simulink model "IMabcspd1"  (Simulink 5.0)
settings: Solver=ode45  StartTime=0.0  StopTime=4.0  RelTol=1e-3
InitFcn:
  | imparamspd1
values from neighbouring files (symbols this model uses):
  Bm = 0.10    (= 0.1)    [IMabc2.m]    (also in imabcparam.m = 0.01; IMabcrun0.m = 0.01; IMabcrun1.m = 0.001; IMcur0.m = 1e-06)
  gam = 2*pi/3    (= 2.09439510239)    [IMabc2.m]    (also in IMabcf0.m; IMabcf1.m; imabcparam.m; IMabcrun0.m)
  J = 0.02    [imabcparam.m]    (also in IMabcrun0.m; IMabcrun1.m; imdefSIvec1.m = 0.03)
  Lm1 = 2/3*Lm    [IMabcf0.m]    (also in IMabcf1.m; imabcparam.m = 0.0564666666667; IMabcrun0.m = 0.0564666666667; IMabcrun1.m = 0.0564666666667)
  Lrr = [Lr   -Lm/2 -Lm/2    [IMabc2.m]    (also in IMabcf0.m = [Lr   -Lm1/2 -Lm1/2; IMabcf1.m = [Lr   -Lm1/2 -Lm1/2)
  Lss = [Ls   -Lm/2 -Lm/2    [IMabc2.m]    (also in IMabcf0.m = [Ls   -Lm1/2 -Lm1/2; IMabcf1.m = [Ls   -Lm1/2 -Lm1/2)
  nsync = 120*freq0/p    (= 1800)    [imabcparam.m]
  p = cos(beta-alpha)    [abcRwdg.m]    (also in alternator.m = 0:pi/20:2*pi; altwdgs.m = 0:pi/20:2*pi; brushlessdcB.m = 0:pi/100:2*pi; brushlessdcnew.m = 0:pi/100:2*pi)
  R = str2num(get(h,'string'))    [acttrcalc1.m]    (also in IMabc2.m = diag([Rs Rs Rs Rr Rr Rr]); IMabcf0.m = diag([Rs Rs Rs Rr Rr Rr]); IMabcf1.m = diag([Rs Rs Rs Rr Rr Rr]); IMcurf0.m = diag([Rs Rs Rr Rr]))
  Vm = Vll*sqrt(2/3)    [imabcparam.m]
  wo = 2*pi*freq0    [calc0.m]    (also in IMabc2.m = 376.991118431; imabcparam.m = 376.991118431; IMabcrun0.m = 376.991118431; IMabcrun1.m = 376.991118431)
undefined symbols (not defined in the file or in its folder): TL1
libraries: simulink x9

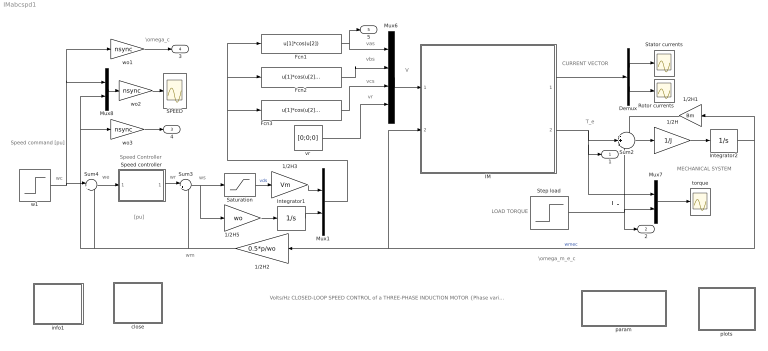
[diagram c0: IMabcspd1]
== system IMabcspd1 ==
  note: LOAD TORQUE
  note: T_L
  note: Volts/Hz CLOSED-LOOP SPEED CONTROL of a THREE-PHASE INDUCTION MOTOR {Phase variable model}
  note: T_e
  note: I
  note: MECHANICAL SYSTEM
  note: \omega_m_e_c
  note: CURRENT VECTOR
  note: V
  note: wr
  note: we
  note: wm
  note: vas
  note: vbs
  note: vcs
  note: vr
  note: Speed command [pu]
  note: \omega_c
  note: [pu]
  note: ws
  note: Speed Controller
  note: wc
  1/2H : Gain  Gain=1/J
  1/2H1 : Gain  Orientation=left  Gain=Bm
  1/2H2 : Gain  Orientation=left  Gain=0.5*p/wo
  1/2H3 : Gain  Gain=Vm
  1/2H5 : Gain  Gain=wo
  Demux : Demux  Outputs=2
  Fcn1 : Fcn  Expr=u[1]*cos(u[2])
  Fcn2 : Fcn  Expr=u[1]*cos(u[2]-gam)
  Fcn3 : Fcn  Expr=u[1]*cos(u[2]+gam)
  IM : Subsystem
  Integrator1 : Integrator
  Integrator2 : Integrator
  Mux1 : Mux  Inputs=2
  Mux6 : Mux
  Mux7 : Mux  Inputs=2
  Mux8 : Mux  Inputs=2
  Rotor currents : Scope
  SPEED : Scope
  Saturation : Saturate  UpperLimit=1  LowerLimit=-1
  Speed controller : Subsystem  mask{Kp=0.6, Ki=5.6, sat=0.03}
      mask prompts: Kp "Proportional gain (Kp)"; Ki "Integral gain (Ki)"; sat "Saturation limit [pu]"
      mask help: Proportional-Integral Speed Controller
  Stator currents : Scope
  Step load : Step  Time=2  Before=0.0  After=TL1  SampleTime=0
  Sum2 : Sum  Inputs=-+-
  Sum3 : Sum  Inputs=|++
  Sum4 : Sum  Inputs=|+-
  close : Subsystem
  info1 : Subsystem
  param : Subsystem
  plots : Subsystem
  torque : Scope
  vr : Constant  Value=[0;0;0]  VectorParams1D=off
  w1 : Step  Time=3  Before=1  After=0.5  SampleTime=0
  wo1 : Gain  Gain=nsync
  wo2 : Gain  Gain=nsync
  wo3 : Gain  Gain=nsync
  1 : Outport
  2 : Outport  Port=2
  4 : Outport  Port=3
  3 : Outport  Port=4
  5 : Outport  Port=5
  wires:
  Demux/1 -> Stator currents/1
  Demux/2 -> Rotor currents/1
  IM/1(I) -> Demux/1
  Sum2/1 -> 1/2H/1
  1/2H/1 -> Integrator2/1
  Integrator2/1 -> 1/2H1/1, IM/2(wmec), 1/2H2/1  "wmec"
  Mux7/1 -> torque/1
  Step load/1 -> Mux7/2, Sum2/3, 2/1
  IM/2(Te) -> Sum2/2, Mux7/1, 1/1
  1/2H1/1 -> Sum2/1
  Sum4/1 -> Speed controller/1(we)
  Mux8/1 -> wo2/1
  Sum3/1 -> Saturation/1, 1/2H5/1
  Speed controller/1(wr) -> Sum3/1
  w1/1 -> Sum4/1, Mux8/1, wo1/1
  Saturation/1 -> 1/2H3/1  "vds"
  1/2H2/1 -> Sum3/2, Sum4/2, Mux8/2, wo3/1
  1/2H3/1 -> Mux1/1
  1/2H5/1 -> Integrator1/1
  Mux6/1 -> IM/1(V)
  Fcn1/1 -> Mux6/1, 5/1
  Fcn2/1 -> Mux6/2
  vr/1 -> Mux6/4
  Mux1/1 -> Fcn1/1, Fcn2/1, Fcn3/1
  Integrator1/1 -> Mux1/2
  wo2/1 -> SPEED/1
  wo3/1 -> 4/1
  wo1/1 -> 3/1
  Fcn3/1 -> Mux6/3

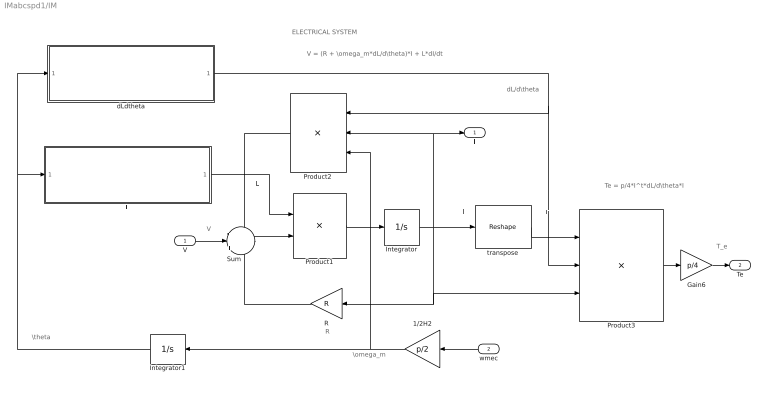
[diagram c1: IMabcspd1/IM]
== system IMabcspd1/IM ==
  note: I
  note: I'
  note: ELECTRICAL SYSTEM
  note: V
  note: \omega_m
  note: \theta
  note: L
  note: T_e
  note: dL/d\theta
  note: R
  note: V = (R + \omega_m*dL/d\theta)*I + L*dI/dt
  note: Te = p/4*I^t*dL/d\theta*I
  V : Inport  PortDimensions=6*1
  wmec : Inport  Orientation=left  Port=2
  1/2H2 : Gain  Orientation=left  Gain=p/2
  Gain6 : Gain  Gain=p/4  ShowAdditionalParam=on
  Integrator : Integrator  InitialCondition=[0 ;0 ;0; 0 ;0 ;0]
  Integrator1 : Integrator  Orientation=left
  L : Subsystem
  Product1 : Product  Inputs=/*  Multiplication=Matrix(*)
  Product2 : Product  Orientation=left  Inputs=3  Multiplication=Matrix(*)
  Product3 : Product  Inputs=3  Multiplication=Matrix(*)  ShowAdditionalParam=on
  R : Gain  Orientation=left  Gain=R  Multiplication=Matrix(K*u)
  Sum : Sum  Inputs=-|+|-
  dLdtheta : Subsystem
  transpose : simulink/Math Operations/Reshape  OutputDimensionality=Row vector  OutputDimensions=[1,6]
  I : Outport
  Te : Outport  Port=2
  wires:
  Product1/1 -> Integrator/1
  Integrator/1 -> Product3/3, R/1, transpose/1, Product2/2, I/1
  Sum/1 -> Product1/2
  R/1 -> Sum/3
  transpose/1 -> Product3/1
  Product2/1 -> Sum/1
  dLdtheta/1(dLdtheta) -> Product3/2, Product2/1
  Product3/1 -> Gain6/1
  1/2H2/1 -> Integrator1/1, Product2/3
  Integrator1/1 -> dLdtheta/1(theta1), L/1(theta)
  L/1(L) -> Product1/1
  V/1 -> Sum/2
  Gain6/1 -> Te/1
  wmec/1 -> 1/2H2/1

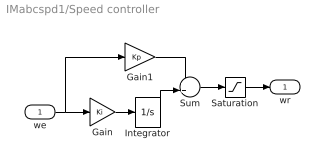
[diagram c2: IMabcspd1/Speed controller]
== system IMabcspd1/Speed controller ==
  we : Inport
  Gain : Gain  Gain=Ki
  Gain1 : Gain  Gain=Kp
  Integrator : Integrator  LimitOutput=on  UpperSaturationLimit=sat  LowerSaturationLimit=-sat
  Saturation : Saturate  UpperLimit=sat  LowerLimit=-sat
  Sum : Sum
  wr : Outport  InitialOutput=0
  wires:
  Saturation/1 -> wr/1
  Sum/1 -> Saturation/1
  Integrator/1 -> Sum/2
  we/1 -> Gain1/1, Gain/1
  Gain/1 -> Integrator/1
  Gain1/1 -> Sum/1

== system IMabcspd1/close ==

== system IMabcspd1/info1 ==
  note: Volts/Hz closed-loop speed control of an induction motor (Phase variable model) [SI]
  note: To modify the machine parameters, double click the block. To adjust the speed controller, double click the PI block. To run the same operation of the induction motor modeled in dq variables, access the file named .

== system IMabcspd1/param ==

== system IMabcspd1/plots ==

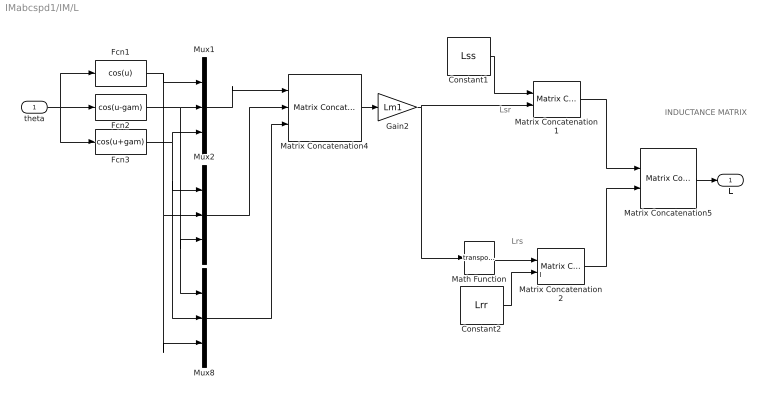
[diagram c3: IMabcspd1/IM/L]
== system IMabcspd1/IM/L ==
  note: L
  note: INDUCTANCE MATRIX
  note: Lsr
  note: Lrs
  theta : Inport
  Constant1 : Constant  Value=Lss  VectorParams1D=off
  Constant2 : Constant  Value=Lrr  VectorParams1D=off
  Fcn1 : Fcn  Expr=cos(u)
  Fcn2 : Fcn  Expr=cos(u-gam)
  Fcn3 : Fcn  Expr=cos(u+gam)
  Gain2 : Gain  Gain=Lm1
  Math Function : Math  Operator=transpose
  Matrix Concatenation1 : simulink/Math Operations/Matrix Concatenation  numInports=2  catMethod=Horizontal
  Matrix Concatenation2 : simulink/Math Operations/Matrix Concatenation  numInports=2  catMethod=Horizontal
  Matrix Concatenation4 : simulink/Math Operations/Matrix Concatenation  numInports=3  catMethod=Horizontal
  Matrix Concatenation5 : simulink/Math Operations/Matrix Concatenation  numInports=2  catMethod=Vertical
  Mux1 : Mux  Inputs=3
  Mux2 : Mux  Inputs=3
  Mux8 : Mux  Inputs=3
  L : Outport
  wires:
  Matrix Concatenation5/1 -> L/1
  theta/1 -> Fcn3/1, Fcn1/1, Fcn2/1
  Math Function/1 -> Matrix Concatenation2/1
  Gain2/1 -> Matrix Concatenation1/2, Math Function/1
  Mux1/1 -> Matrix Concatenation4/1
  Matrix Concatenation4/1 -> Gain2/1
  Mux8/1 -> Matrix Concatenation4/3
  Mux2/1 -> Matrix Concatenation4/2
  Matrix Concatenation1/1 -> Matrix Concatenation5/1
  Matrix Concatenation2/1 -> Matrix Concatenation5/2
  Constant1/1 -> Matrix Concatenation1/1
  Constant2/1 -> Matrix Concatenation2/2
  Fcn3/1 -> Mux1/3, Mux2/1, Mux8/2
  Fcn2/1 -> Mux1/2, Mux2/3, Mux8/1
  Fcn1/1 -> Mux8/3, Mux2/2, Mux1/1

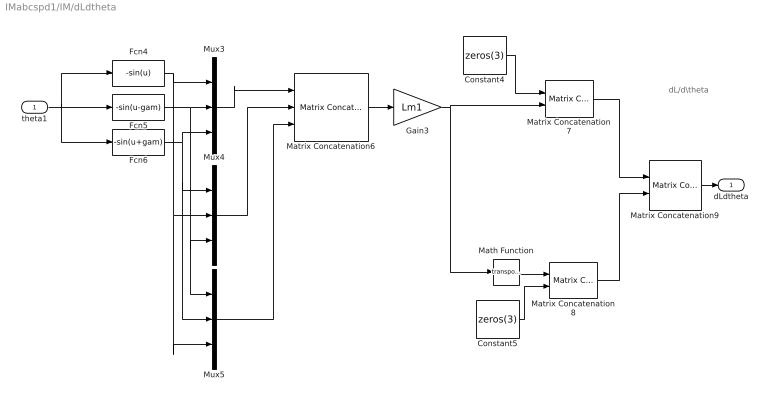
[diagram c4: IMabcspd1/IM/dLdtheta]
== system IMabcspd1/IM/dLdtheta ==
  note: dL/d\theta
  theta1 : Inport
  Constant4 : Constant  Value=zeros(3)  VectorParams1D=off
  Constant5 : Constant  Value=zeros(3)  VectorParams1D=off
  Fcn4 : Fcn  Expr=-sin(u)
  Fcn5 : Fcn  Expr=-sin(u-gam)
  Fcn6 : Fcn  Expr=-sin(u+gam)
  Gain3 : Gain  Gain=Lm1
  Math Function : Math  Operator=transpose
  Matrix Concatenation6 : simulink/Math Operations/Matrix Concatenation  numInports=3  catMethod=Horizontal
  Matrix Concatenation7 : simulink/Math Operations/Matrix Concatenation  numInports=2  catMethod=Horizontal
  Matrix Concatenation8 : simulink/Math Operations/Matrix Concatenation  numInports=2  catMethod=Horizontal
  Matrix Concatenation9 : simulink/Math Operations/Matrix Concatenation  numInports=2  catMethod=Vertical
  Mux3 : Mux  Inputs=3
  Mux4 : Mux  Inputs=3
  Mux5 : Mux  Inputs=3
  dLdtheta : Outport
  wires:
  Matrix Concatenation9/1 -> dLdtheta/1
  theta1/1 -> Fcn5/1, Fcn4/1, Fcn6/1
  Gain3/1 -> Matrix Concatenation7/2, Math Function/1
  Mux4/1 -> Matrix Concatenation6/2
  Mux3/1 -> Matrix Concatenation6/1
  Matrix Concatenation6/1 -> Gain3/1
  Mux5/1 -> Matrix Concatenation6/3
  Matrix Concatenation7/1 -> Matrix Concatenation9/1
  Matrix Concatenation8/1 -> Matrix Concatenation9/2
  Constant4/1 -> Matrix Concatenation7/1
  Constant5/1 -> Matrix Concatenation8/2
  Fcn6/1 -> Mux3/3, Mux4/1, Mux5/2
  Fcn5/1 -> Mux3/2, Mux4/3, Mux5/1
  Fcn4/1 -> Mux3/1, Mux4/2, Mux5/3
  Math Function/1 -> Matrix Concatenation8/1
